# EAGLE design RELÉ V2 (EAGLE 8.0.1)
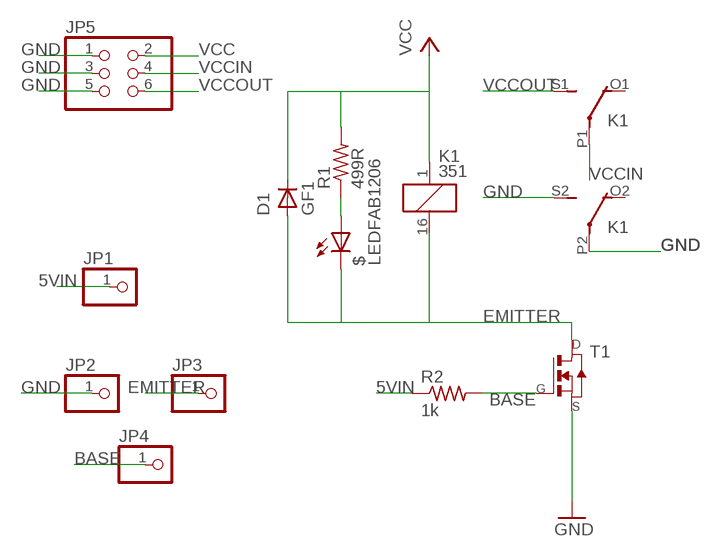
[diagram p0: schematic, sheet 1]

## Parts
$  LEDFAB1206  [LED1206FAB]
D1  GF1  [SMA-DO214AC]
JP1  PINHD-1X1  [1X01]
JP2  PINHD-1X1  [1X01]
JP3  PINHD-1X1  [1X01]
JP4  PINHD-1X1  [1X01]
JP5  PINHD-2X3-SMD  [2X03SMD]
K1  351  [351]
R1  499R  RES-US1206FAB  [R1206FAB]
R2  1k  RES-US1206FAB  [R1206FAB]
T1  NMOSFETSOT23  [SOT-23]

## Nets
5VIN: JP1.1 R2.1
BASE: JP4.1 R2.2 T1.3(G)
EMITTER: $.2(C) D1.A JP3.1 K1.16 T1.1(D)
GND: JP2.1 JP5.1 JP5.3 JP5.5 K1.P2(3:P) K1.S2(3:S) T1.2(S)
N$1: $.1(A) R1.1
VCC: D1.K(C) JP5.2 K1.1 R1.2
VCCIN: JP5.4 K1.P1(2:P)
VCCOUT: JP5.6 K1.S1(2:S)
Unconnected: K1.O1(2:O) K1.O2(3:O)

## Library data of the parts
$ = fab:LED: LED
D1 = diode:GF1: DIODE
JP1-JP4 = pinhead:PINHD-1X1: PIN HEADER
JP5 = fab:PINHD-2X3-SMD: PIN HEADER
K1 = relay:351: RELAY 2 x switch, Omron; OC_FARNELL: unknown; OC_NEWARK: unknown
R1 R2 = fab:RES-US: Resistor (US Symbol)
T1 = fab:NMOSFET: MOS FET

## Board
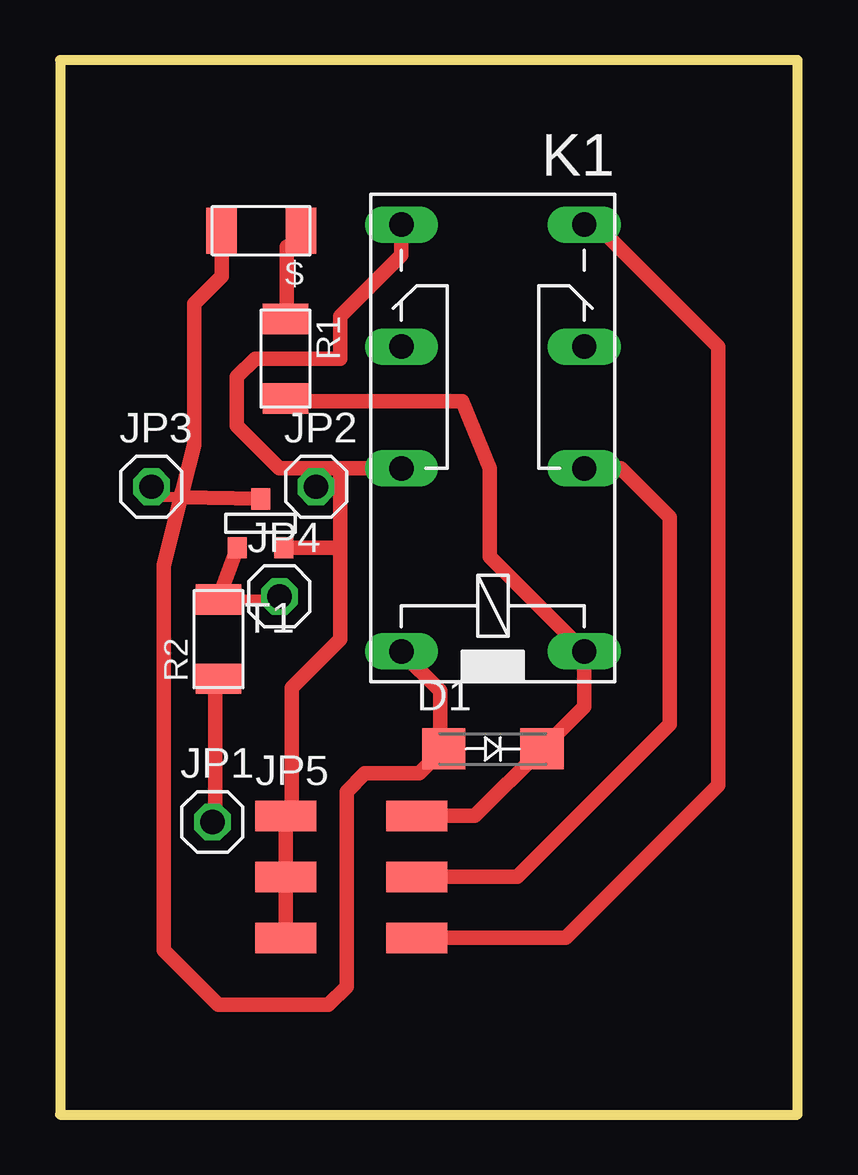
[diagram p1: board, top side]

Size 30.73 x 43.94 mm. Coordinates in mm from the lower left corner, seen from the top.
Outline: 0,0 30.73,0 30.73,43.94 0,43.94 0,0
Copper layers (1*16): Top 0.035mm / dielectric 1.5mm / Bottom 0.035mm
Design rules "default": minimum track width 10mil, minimum drill 24mil, track to track 8mil, track to pad 8mil, pad to pad 8mil, via to via 8mil, smd to smd 8mil, copper to edge 40mil, drill to drill 8mil, minimum pad ring 10mil, minimum via ring 8mil, stop-mask expansion 4mil, vias tented up to drill 0mil, thermal gap 10mil

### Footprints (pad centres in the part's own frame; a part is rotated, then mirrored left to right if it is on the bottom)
LED1206FAB = smd 1.27 x 1.905: 1 -1.651,0; 2 1.651,0
SMA-DO214AC = smd 1.8 x 1.7: A -2.05,0; K 2.05,0
1X01 = drill 1.016 octagon: 1 0,0
2X03SMD = smd 2.54 x 1.27: 1 -2.54,2.54; 2 2.92,2.54; 3 -2.54,0; 4 2.92,0; 5 -2.54,-2.54; 6 2.92,-2.54
351 = drill 1.016 long: 1 -3.81,-3.81; 16 -3.81,3.81; O1 8.89,-3.81; O2 8.89,3.81; P1 3.81,-3.81; P2 3.81,3.81; S1 13.97,-3.81; S2 13.97,3.81
R1206FAB = smd 1.27 x 1.905: 1 -1.651,0; 2 1.651,0
SOT-23 = smd 0.787 x 0.889: 1 0.025,-1.016; 2 -0.94,1.016; 3 0.991,1.016

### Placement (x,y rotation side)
$  8.38,36.83 180 top
D1  18.03,15.24 0 top
JP1  6.35,12.19 0 top
JP2  10.67,26.16 0 top
JP3  3.81,26.16 0 top
JP4  9.14,21.59 0 top
JP5  11.94,9.91 0 top
K1  18.03,23.11 90 top
R1  9.4,31.5 270 top
R2  6.6,19.81 90 top
T1  8.38,24.64 180 top

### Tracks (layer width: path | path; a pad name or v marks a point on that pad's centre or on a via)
5VIN
  Top 0.254: 6.48,18.11 R2.1 | 6.48,12.39 JP1.1
  Top 0.61: 6.48,12.39 6.48,18.11
BASE
  Top 0.406: R2.2 9.14,21.46 JP4.1
  Top 0.61: T1.3 R2.2
EMITTER
  Top 0.254: D1.A 15.85,15.37 | 14.25,19.25 K1.16
  Top 0.406: 5.04,25.73 3.81,25.73 JP3.1
  Top 0.61: 15.85,15.37 15.85,17.65 14.25,19.25 | $.2 6.73,34.92 5.59,33.78 5.59,27.91 5.11,26.03 5.04,25.73 | 16,15.22 D1.A 14.97,14.22 12.7,14.22 11.94,13.46 11.94,5.33 11.18,4.57 6.6,4.57 4.32,6.86 4.32,22.86 5.04,25.73 | T1.1 5.04,25.73
GND
  Top 0.61: 11.68,23.62 11.68,26.92 | 11.68,23.62 11.68,19.81 9.65,17.78 9.65,12.7 JP5.1 JP5.3 JP5.5 | K1.S2 14.22,35.81 11.68,33.27 11.68,31.5 8.13,31.5 7.37,30.73 7.37,28.7 9.14,26.92 10.67,26.92 | 10.67,26.92 11.68,26.92 | T1.2 11.68,23.62 | JP2.1 10.67,26.92 | K1.P2 11.68,26.92
N$1
  Top 0.254: 9.91,36.63 9.45,36.17 | 9.45,33.2 R1.1
  Top 0.61: 9.45,36.17 9.45,33.2 | 9.91,36.63 $.1
N$3  (1 unrouted)
VCC
  Top 0.61: R1.2 9.53,29.72 16.76,29.72 17.91,26.92 17.91,23.24 K1.1 21.84,17 D1.K 17.29,12.45 JP5.2
VCCIN
  Top 0.61: K1.P1 23.37,26.92 25.4,24.89 25.4,16.26 19.05,9.91 JP5.4
VCCOUT
  Top 0.61: K1.S1 22.35,37.08 27.43,32 27.43,13.72 21.08,7.37 JP5.6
